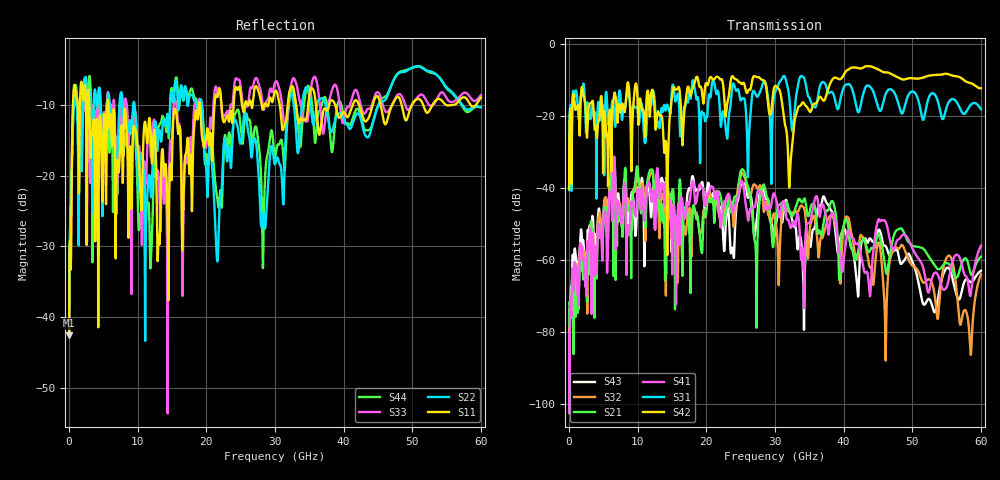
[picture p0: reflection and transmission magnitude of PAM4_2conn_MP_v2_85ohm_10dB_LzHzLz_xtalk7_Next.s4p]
! Info: Touchstone file created by Circ.  Input file=FAB50GbE_2conn_Midplane_Examax_Topo2_v2_85ohm_10dB_LzHzLz.circ
# Hz S RI R 50
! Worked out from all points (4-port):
!   6000 points, 10 MHz to 60 GHz, reference 50 ohm
!   strongest paths, dB at 10 MHz, 15.01 GHz, 30.01 GHz, 45.01 GHz, 60 GHz:
!     S42: -40.3, -14.5, -11.7, -7.0, -12.3
!     S31: -40.6, -12.2, -13.6, -17.5, -18.1
!     S41: -88.0, -61.6, -42.1, -49.0, -56.1
!     S21: -75.6, -40.9, -50.4, -52.8, -59.1
!     S32: -82.5, -44.8, -47.9, -55.3, -64.1
!     S43: -77.3, -52.0, -51.8, -52.0, -63.0
!   lowest |S11| = -42.6 dB at 10 MHz (marker M1), VSWR 1.02, Z = 50.7 + j0.0453 ohm
!   |S11| at or under -10 dB: 2.948 GHz to 5.582 GHz (2.634 GHz wide, 61.8 % of centre); 5.722 GHz to 18.9 GHz (13.18 GHz wide, 107 % of centre); 38.77 GHz to 41.33 GHz (2.561 GHz wide, 6.39 % of centre)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
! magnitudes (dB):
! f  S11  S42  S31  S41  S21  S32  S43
! 10 MHz  -42.6  -40.3  -40.6  -88.0  -75.6  -82.5  -77.3
! 870 MHz  -7.5  -17.7  -14.2  -63.4  -67.4  -62.1  -57.1
! 11.98 GHz  -16.5  -13.7  -17.0  -43.6  -35.0  -36.0  -47.9
! 15.52 GHz  -10.7  -12.7  -16.0  -53.3  -53.0  -55.7  -52.4
! 25.27 GHz  -10.3  -11.0  -15.1  -38.3  -34.8  -35.9  -38.7
! 32.17 GHz  -7.9  -36.6  -16.6  -50.5  -46.6  -46.9  -46.7
! 60 GHz  -9.0  -12.3  -18.1  -56.1  -59.1  -64.1  -63.0
